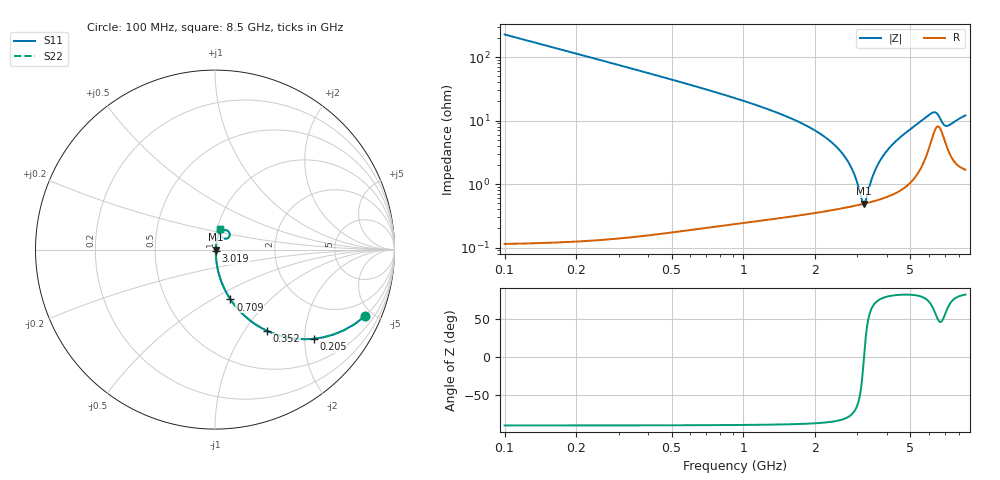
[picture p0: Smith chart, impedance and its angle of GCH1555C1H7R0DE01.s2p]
!Murata Part Number: GCH1555C1H7R0DE01
!These Parameters are Measured in Series Mode Connection
!Data Generated on Mar 13, 2026
!  o--ll--o
!Port1  Port2
!  o------o
!Operation Temp=25[degC], DC Bias Voltage=0[V]
!Freq. Start=100[MHz] Stop=9[GHz] 401[Steps]
# Hz S RI R 50
!Freq.(Hz) S11(Real) S11(Imag) S21(Real) S21(Imag) S12(Real) S12(Imag) S22(Real) S22(Imag)
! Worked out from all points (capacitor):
!   401 points, 100 MHz to 8.5 GHz, reference 50 ohm
!   read as one part in series: C = 7 pF near 142 MHz
!   lowest |Z| = 491 mohm at 3.187 GHz (marker M1)
!   series resonance near 3.199 GHz, so ESL is about 350 pH
!   S11 on the Smith chart (normalised r, x): 100 MHz: 1.00, -4.54; 205 MHz: 1.00, -2.21; 352 MHz: 1.00, -1.28; 709 MHz: 1.00, -0.61; 3.019 GHz: 1.01, -0.02; 8.5 GHz: 1.03, +0.24
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1e8  0.8375 -0.3687  0.1625 0.3687  0.1625 0.3687  0.8375 -0.3687
2.05e8  0.5493 -0.497  0.4507 0.497  0.4507 0.497  0.5493 -0.497
3.52e8  0.2894 -0.4524  0.7106 0.4524  0.7106 0.4524  0.2894 -0.4524
4.99e8  0.1656 -0.3698  0.8344 0.3698  0.8344 0.3698  0.1656 -0.3698
7.09e8  0.0863 -0.2775  0.9137 0.2775  0.9137 0.2775  0.0863 -0.2775
1.507e9  0.0164 -0.1149  0.9836 0.1149  0.9836 0.1149  0.0164 -0.1149
2.431e9  0.0055 -0.0393  0.9945 0.0393  0.9945 0.0393  0.0055 -0.0393
2.704e9  0.00483 -0.0239  0.9952 0.0239  0.9952 0.0239  0.00483 -0.0239
2.914e9  0.00469 -0.0133  0.9953 0.0133  0.9953 0.0133  0.00469 -0.0133
3.019e9  0.00471 -0.00824  0.9953 0.00824  0.9953 0.00824  0.00471 -0.00824
3.124e9  0.00479 -0.00337  0.9952 0.00337  0.9952 0.00337  0.00479 -0.00337
3.187e9  0.00486 -0.000515  0.9951 0.000515  0.9951 0.000515  0.00486 -0.000515
3.25e9  0.00495 0.00229  0.9951 -0.00229  0.9951 -0.00229  0.00495 0.00229
3.46e9  0.00538 0.0113  0.9946 -0.0113  0.9946 -0.0113  0.00538 0.0113
3.649e9  0.00592 0.0191  0.9941 -0.0191  0.9941 -0.0191  0.00592 0.0191
3.922e9  0.00697 0.0298  0.993 -0.0298  0.993 -0.0298  0.00697 0.0298
4.3e9  0.00899 0.0442  0.991 -0.0442  0.991 -0.0442  0.00899 0.0442
5.707e9  0.0322 0.0986  0.9678 -0.0986  0.9678 -0.0986  0.0322 0.0986
6.337e9  0.0767 0.0994  0.9233 -0.0994  0.9233 -0.0994  0.0767 0.0994
6.883e9  0.056 0.0609  0.944 -0.0609  0.944 -0.0609  0.056 0.0609
7.114e9  0.0416 0.0672  0.9584 -0.0672  0.9584 -0.0672  0.0416 0.0672
8.5e9  0.0299 0.1139  0.9701 -0.1139  0.9701 -0.1139  0.0299 0.1139
